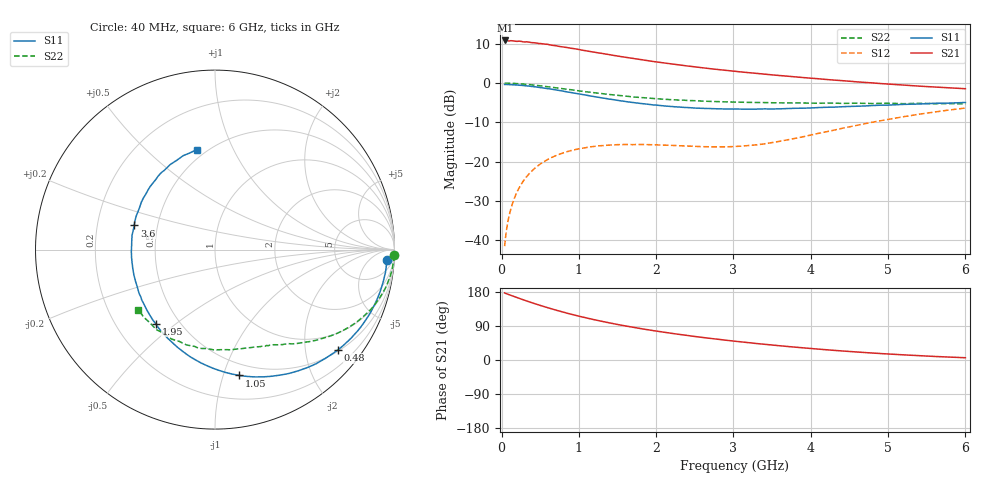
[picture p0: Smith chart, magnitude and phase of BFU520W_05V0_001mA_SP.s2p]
! Filename:  P:\Prog\Test\Noise\ATS_data\Testdata_Net\Run2\BFU520W_APM2013_06_A05_05p0V_001mA_SP_CM01_D.s2p
! Date/Time: Tue 26/Mar/2013 18:01:39
! BFU520W_APM2013_06_A05_05p0V_1to20mA_SP_CM01_Bias1_R.s2p
! MDIF S-parameter v. bias file
! BFU520W_APM2013_06_A05_05p0V_1to20mA_SP_CM01
! Date/time Thu Mar 21 14:22:37 2013
! bias mode 1
! bias variable = I_out
! VAR bias_var= 1
! VAR V_out= 5.0000
! VAR I_out= 0.9950
! VAR V_in= 0.7935
! VAR I_in= 0.0109
! Device data file deembeded for feedlines and parallel
! Original file: \Run2\BFU520W_APM2013_06_A05_05p0V_001mA_SP_CM01_R.s2p
! Feed-files: PR019V01_070313_Feed1.s2p, PR019V01_070313_Feed2.s2p
! Parallel-file: PR019V01_070313_Par.s2p
# MHz S MA R 50
!  Freq-MHz  S11-mag  S11-arg  S21-mag  S21-arg  S12-mag  S12-arg  S22-mag  S22-arg
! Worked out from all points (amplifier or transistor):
!   98 points, 40 MHz to 6 GHz, reference 50 ohm
!   highest |S21| = 10.9 dB at 50 MHz (marker M1)
!   |S21| within 3 dB of that: start of sweep to 1.205 GHz
!   unconditionally stable (mu >= 1): 2.766 GHz to 3.762 GHz
!   at 300 MHz: K = 0.12, MSG = 17.5 dB, |S12| = -24.5 dB
!   at 1.6 GHz: K = 0.57, MSG = 11.1 dB, |S12| = -15.7 dB
!   at 6 GHz: K = 0.81, MSG = 2.5 dB, |S12| = -6.4 dB
!   S11 on the Smith chart (normalised r, x): 40 MHz: 16, -23; 480 MHz: 0.53, -2.72; 1.05 GHz: 0.40, -1.13; 1.95 GHz: 0.37, -0.43; 3.6 GHz: 0.37, +0.13; 6 GHz: 0.45, +0.73
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40  0.9596 -3.4  3.482 177.1  0.008351 87.5  0.9984 -1.9
50  0.9594 -4.2  3.494 176.0  0.01036 87.0  0.9971 -2.3
100  0.9568 -8.4  3.444 172.2  0.02073 84.2  0.9952 -4.7
120  0.9548 -10.2  3.471 170.8  0.0248 83.1  0.9943 -5.6
200  0.9451 -16.8  3.402 164.8  0.0408 78.7  0.9849 -9.3
240  0.938 -20.2  3.417 161.8  0.04847 76.7  0.979 -11.1
340  0.9189 -28.3  3.342 154.8  0.06673 71.6  0.96 -15.5
480  0.8834 -39.2  3.198 145.4  0.08978 65.0  0.929 -21.1
600  0.8496 -48.5  3.114 137.9  0.1066 59.8  0.8979 -25.5
700  0.8185 -55.7  3 131.9  0.1187 55.8  0.872 -28.9
850  0.772 -66.1  2.837 123.5  0.1337 50.5  0.8338 -33.4
1050  0.7141 -79.1  2.622 113.3  0.1481 44.6  0.7846 -38.7
1250  0.6602 -91.2  2.429 104.1  0.1583 39.7  0.7446 -43.1
1500  0.6033 -105.4  2.213 93.8  0.1642 35.0  0.699 -48.3
1950  0.5286 -128.7  1.893 78.0  0.164 30.7  0.6385 -56.1
2050  0.5183 -133.5  1.835 74.9  0.1626 30.6  0.6273 -57.7
2500  0.4806 -154.1  1.61 62.1  0.1562 32.2  0.5966 -65.0
3100  0.4662 -178.7  1.387 47.8  0.1571 43.1  0.5709 -75.4
3600  0.4696 163.3  1.247 37.5  0.1814 53.6  0.5599 -84.9
4100  0.4878 147.4  1.135 28.7  0.2289 59.2  0.5535 -95.4
5200  0.5354 117.9  0.9439 13.6  0.3729 55.5  0.5463 -121.0
6000  0.5662 100.4  0.8484 6.0  0.4807 46.3  0.5422 -141.8
